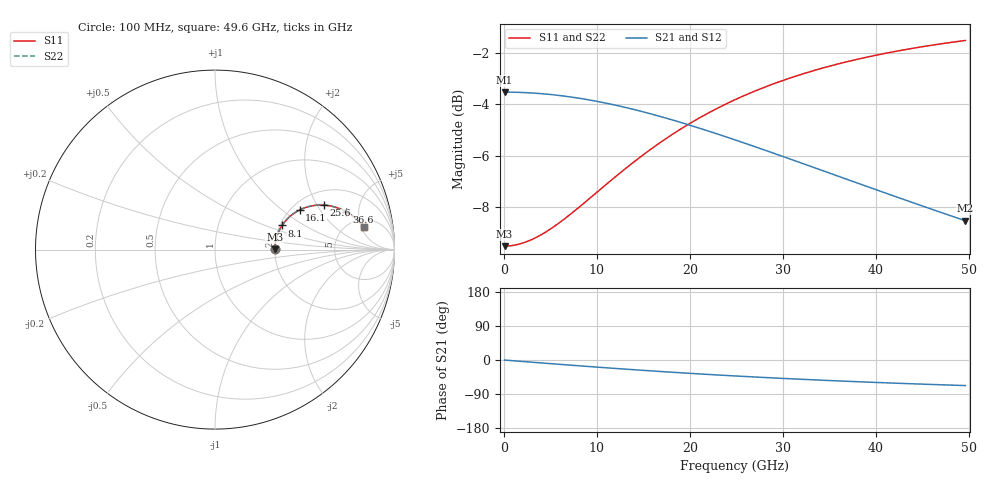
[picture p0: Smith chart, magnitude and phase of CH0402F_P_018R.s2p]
# GHz S RI R 18
! S-Parameters data
! Freq  reS11  imS11  reS21  imS21  reS12  imS12  reS22  imS22
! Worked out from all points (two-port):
!   100 points, 100 MHz to 49.6 GHz, reference 18 ohm
!   highest |S21| = -3.52 dB at 100 MHz (marker M1); lowest = -8.5 dB at 49.6 GHz (marker M2)
!   |S21| within 3 dB of the highest: start of sweep to 33.74 GHz
!   lowest |S11| = -9.5 dB at 100 MHz (marker M3), VSWR 2.00, Z = 36 + j0.144 ohm
!   |S11| at or under -10 dB: nowhere
!   |S22| runs from -9.5 to -1.5 dB; largest |S21 - S12| = 0
!   S11 on the Smith chart (normalised r, x): 100 MHz: 2.00, +0.01; 8.1 GHz: 2.05, +0.66; 16.1 GHz: 2.22, +1.34; 25.6 GHz: 2.63, +2.28; 36.6 GHz: 3.63, +3.63; 49.6 GHz: 6.72, +5.68
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0.1  0.3333 0.00178  0.6667 -0.00223  0.6667 -0.00223  0.3333 0.00178
1.6  0.335 0.0284  0.665 -0.0356  0.665 -0.0356  0.335 0.0284
3.6  0.3417 0.0632  0.6582 -0.0795  0.6582 -0.0795  0.3417 0.0632
5.6  0.3532 0.0964  0.6465 -0.1217  0.6465 -0.1217  0.3532 0.0964
8.1  0.3738 0.1345  0.6256 -0.1711  0.6256 -0.1711  0.3738 0.1345
8.6  0.3786 0.1415  0.6206 -0.1804  0.6206 -0.1804  0.3786 0.1415
10.6  0.4 0.1677  0.5988 -0.2156  0.5988 -0.2156  0.4 0.1677
12.6  0.4242 0.1903  0.5742 -0.2472  0.5742 -0.2472  0.4242 0.1903
14.1  0.4437 0.2047  0.5542 -0.2684  0.5542 -0.2684  0.4437 0.2047
16.1  0.4711 0.2206  0.5263 -0.2933  0.5263 -0.2933  0.4711 0.2206
16.6  0.4781 0.2239  0.5191 -0.2989  0.5191 -0.2989  0.4781 0.2239
18.6  0.5065 0.2351  0.49 -0.3191  0.49 -0.3191  0.5065 0.2351
20.6  0.5351 0.2427  0.4606 -0.3357  0.4606 -0.3357  0.5351 0.2427
22.6  0.5634 0.247  0.4314 -0.349  0.4314 -0.349  0.5634 0.247
25.1  0.5978 0.2481  0.3957 -0.3613  0.3957 -0.3613  0.5978 0.2481
25.6  0.6046 0.2478  0.3888 -0.3633  0.3888 -0.3633  0.6046 0.2478
29.1  0.6497 0.2417  0.3417 -0.3728  0.3417 -0.3728  0.6497 0.2417
33.1  0.6964 0.2273  0.2925 -0.3762  0.2925 -0.3762  0.6964 0.2273
36.6  0.7326 0.2098  0.2538 -0.3743  0.2538 -0.3743  0.7326 0.2098
41.6  0.7771 0.1795  0.2054 -0.3661  0.2054 -0.3661  0.7771 0.1795
45.6  0.8068 0.1523  0.1721 -0.3565  0.1721 -0.3565  0.8068 0.1523
49.6  0.8319 0.1236  0.1432 -0.3452  0.1432 -0.3452  0.8319 0.1236
